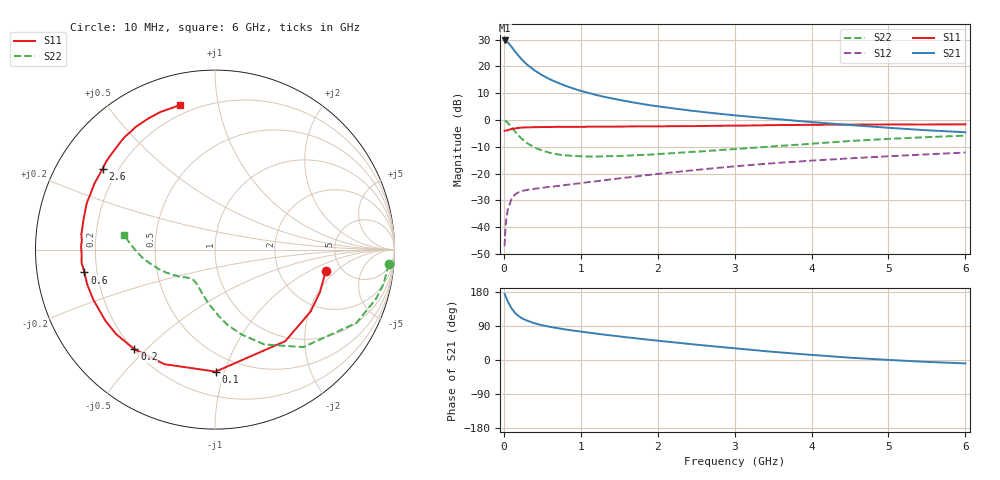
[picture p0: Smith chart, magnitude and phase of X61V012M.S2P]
! SIEMENS Small Signal Semiconductors
! BFP193W
! Si NPN RF Bipolar Junction Transistor in SOT343
! VCE = 1 V  IC = 12 mA
! Common Emitter S-Parameters:  April 1994
# GHz  S  MA  R  50
!  f  S11  S21  S12  S22
! GHz  MAG  ANG  MAG  ANG  MAG  ANG  MAG  ANG
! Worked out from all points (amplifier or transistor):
!   40 points, 10 MHz to 6 GHz, reference 50 ohm
!   highest |S21| = 29.7 dB at 10 MHz (marker M1)
!   |S21| within 3 dB of that: start of sweep to 116.4 MHz
!   unconditionally stable (mu >= 1): 1.13 GHz to 5.735 GHz
!   at 200 MHz: K = 0.26, MSG = 25.3 dB, |S12| = -26.9 dB
!   at 1.5 GHz: K = 1.12, MAG = 12.6 dB, |S12| = -21.8 dB
!   at 6 GHz: K = 0.99, MSG = 3.8 dB, |S12| = -12.1 dB
!   S11 on the Smith chart (normalised r, x): 10 MHz: 3.75, -1.49; 100 MHz: 0.37, -0.93; 200 MHz: 0.20, -0.46; 600 MHz: 0.15, -0.08; 2.6 GHz: 0.14, +0.32; 6 GHz: 0.15, +0.78
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0.01  0.6283 -11.0  30.59 174.0  0.0044 83.8  0.971 -4.9
0.02  0.631 -22.1  30.42 169.6  0.0092 79.7  0.9584 -11.5
0.03  0.6348 -32.9  29.96 164.6  0.0133 75.8  0.9386 -16.9
0.05  0.6431 -52.5  28.34 154.9  0.0208 67.8  0.8884 -27.3
0.1  0.6797 -89.7  23.25 136.3  0.0338 52.2  0.733 -47.8
0.15  0.6978 -113.8  18.71 123.3  0.0411 42.3  0.596 -62.5
0.2  0.714 -129.0  15.23 114.8  0.0453 37.3  0.495 -72.7
0.25  0.7248 -139.5  12.8 108.6  0.0478 34.0  0.4253 -80.6
0.3  0.7281 -147.0  10.88 104.0  0.0494 32.1  0.3712 -86.7
0.4  0.7333 -157.6  8.421 96.9  0.0519 30.7  0.306 -96.2
0.5  0.738 -164.8  6.842 91.6  0.0542 31.2  0.268 -103.3
0.6  0.7386 -170.1  5.742 87.5  0.0565 31.9  0.2436 -109.0
0.8  0.7434 -178.1  4.359 80.7  0.061 34.7  0.2189 -116.8
1.1  0.7498 173.5  3.207 72.3  0.0691 38.6  0.2078 -125.0
1.3  0.7501 168.6  2.72 67.0  0.0748 40.8  0.2095 -128.5
1.6  0.756 162.4  2.236 59.8  0.0842 43.6  0.2155 -132.9
2.2  0.7659 151.3  1.65 46.8  0.1055 45.7  0.2402 -141.0
2.6  0.7715 144.3  1.404 38.5  0.1205 45.9  0.2609 -146.4
3.2  0.7894 134.6  1.152 27.2  0.1439 44.4  0.2997 -154.6
4.5  0.8196 116.9  0.806 6.1  0.1922 38.0  0.405 -173.2
5.5  0.8245 107.8  0.643 -5.0  0.2282 32.5  0.4783 175.5
6  0.8288 103.5  0.59 -8.9  0.2469 29.8  0.5106 171.0
